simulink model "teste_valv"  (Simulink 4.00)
settings: Solver=ode45  StartTime=0.0  StopTime=8  RelTol=1e-3
libraries: simulink3 x1

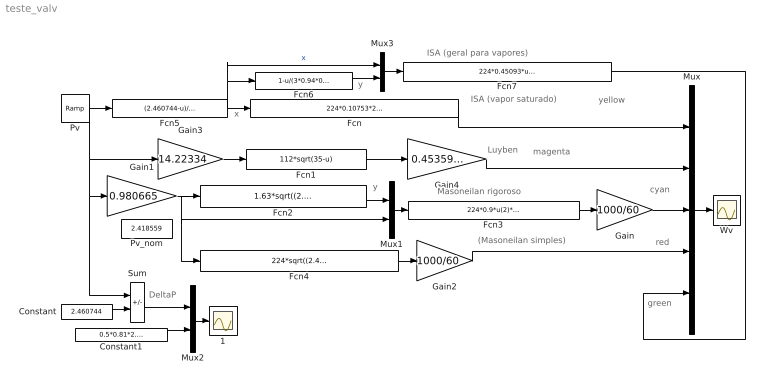
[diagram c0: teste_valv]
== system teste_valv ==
  note: y
  note: x
  note: yellow
  note: magenta
  note: cyan
  note: red
  note: (Masoneilan simples)
  note: Masoneilan rigoroso
  note: Luyben
  note: ISA (vapor saturado)
  note: DeltaP
  note: y
  note: ISA (geral para vapores)
  note: green
  1 : Scope
  Constant : Constant  Value=2.460744
  Constant1 : Constant  Value=0.5*0.81*2.460744
  Fcn : Fcn  Expr=224*0.10753*2.460744*(3-u/0.6804)*sqrt(u)
  Fcn1 : Fcn  Expr=112*sqrt(35-u)
  Fcn2 : Fcn  Expr=1.63*sqrt((2.413165-u)/2.413165)/0.9
  Fcn3 : Fcn  Expr=224*0.9*u(2)*(u(1)-0.148*u(1)^3)/83.7
  Fcn4 : Fcn  Expr=224*sqrt((2.413165-u)*(2.413165+u))/72.4
  Fcn5 : Fcn  Expr=(2.460744-u)/2.460744
  Fcn6 : Fcn  Expr=1-u/(3*0.94*0.6804)
  Fcn7 : Fcn  Expr=224*0.45093*u(2)*sqrt(u(1)*2.460744*1.62087)
  Gain : Gain  Gain=1000/60  Multiplication=Element-wise(K.*u)  SaturateOnIntegerOverflow=on
  Gain1 : Gain  Gain=0.980665  Multiplication=Element-wise(K.*u)  SaturateOnIntegerOverflow=on
  Gain2 : Gain  Gain=1000/60  Multiplication=Element-wise(K.*u)  SaturateOnIntegerOverflow=on
  Gain3 : Gain  Gain=14.22334  Multiplication=Element-wise(K.*u)  SaturateOnIntegerOverflow=on
  Gain4 : Gain  Gain=0.4535924  Multiplication=Element-wise(K.*u)  SaturateOnIntegerOverflow=on
  Mux : Mux  Inputs=5
  Mux1 : Mux  Inputs=2
  Mux2 : Mux  Inputs=2
  Mux3 : Mux  Inputs=2
  Pv : simulink3/Sources/Ramp  slope=0.1  start=0  X0=1.5
  Pv_nom : Constant  Value=2.418559
  Sum : Sum  Inputs=-+  SaturateOnIntegerOverflow=on
  Wv : Scope
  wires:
  Pv/1 -> Fcn5/1, Gain3/1, Gain1/1, Sum/1
  Fcn/1 -> Mux/1
  Mux/1 -> Wv/1
  Mux1/1 -> Fcn3/1
  Fcn3/1 -> Gain/1
  Gain1/1 -> Fcn2/1, Fcn4/1, Mux1/2
  Fcn1/1 -> Gain4/1
  Fcn4/1 -> Gain2/1
  Fcn5/1 -> Fcn/1, Fcn6/1, Mux3/1  "x"
  Gain3/1 -> Fcn1/1
  Gain4/1 -> Mux/2
  Gain/1 -> Mux/3
  Gain2/1 -> Mux/4
  Constant/1 -> Sum/2
  Sum/1 -> Mux2/1
  Mux2/1 -> 1/1
  Constant1/1 -> Mux2/2
  Fcn2/1 -> Mux1/1
  Fcn6/1 -> Mux3/2
  Mux3/1 -> Fcn7/1
  Fcn7/1 -> Mux/5
